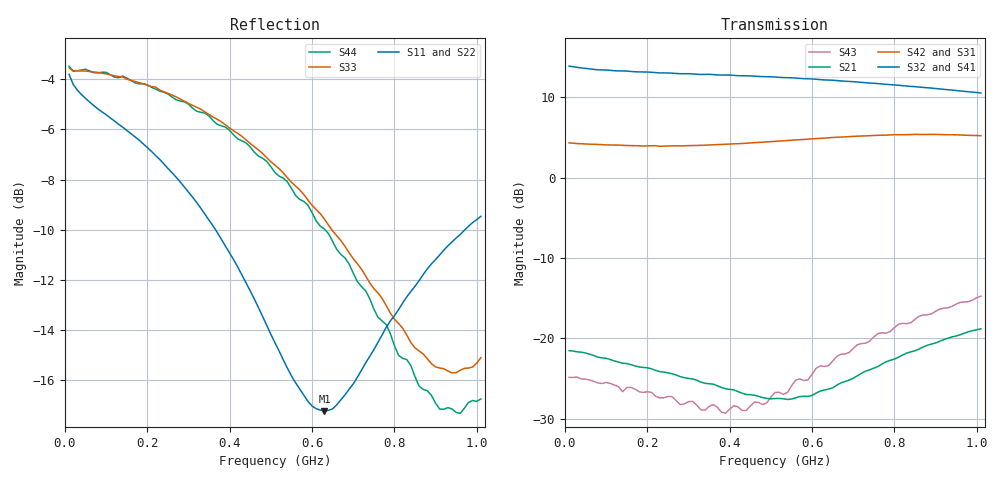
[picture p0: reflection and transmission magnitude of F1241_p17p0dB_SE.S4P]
! Integrated Device Technology
! Corporate Headquarters
! 6024 Silver Creek Valley Road
! San Jose, CA 95138  USA
! Phone:  1-408-284-8200
! Toll Free:  1-800-223-1366
! Webpage:  http://www.idt.com/
! Timing and RF Division
! 515 Groton Road, Suite 102
! Westford, MA 01886-6024
! Device:  F1241
! Description: Dual Intermediate Frequency Digital Variable Gain Amplifier
! Frequency:  10.0 -  500.00 MHz
! Package:  5x5 mm QFN Plastic Package: 32 pin
! Ports:  8 RF, 20 DC
!  Pin  1  = GA3  Pin 17  = RF OUT_B+
!  Pin  2  = GA4  Pin 18  = RF OUT_B-
!  Pin  3  = GA5  Pin 19  = STBY_B
!  Pin  4  = ISET_A  Pin 20  = Ground
!  Pin  5  = ISET_B  Pin 21  = Ground
!  Pin  6  = GB5  Pin 22  = STB_A
!  Pin  7  = GB4  Pin 23  = RF OUT_A-  = Port 4
!  Pin  8  = GB3  Pin 24  = RF OUT_A+  = Port 3
!  Pin  9  = GB2  Pin 25  = NO CONNECT
!  Pin 10  = GB1  Pin 26  = NO CONNECT
!  Pin 11  = RF IN_B+  Pin 27  = VCC
!  Pin 12  = RF IN_B-  Pin 28  = Ground
!  Pin 13  = Ground  Pin 29  = RF IN_A-  = Port 2
!  Pin 14  = VCC  Pin 30  = RF IN_A+  = Port 1
!  Pin 15  = NO CONNECT  Pin 31  = GA1
!  Pin 16  = NO CONNECT  Pin 32  = GA2
! State:  3
! Gain State:  17.0 dB
! Voltages:  Vcc = +5.00 Volts  Icc approximately 160.0 mA or 80 mA per channel.
! Data:  The device was measured on a custom evaluation board which has
!  individual transmission lines to the RF pins.  Data was collected
!  using a calibrated network analyzer.  The evaluation board was
!  de-embedded using a port reference technique.
!  The reference plane is the edge of the package pin.
!  Only Channel A was measured.
!  This data is in single-ended operation.  If your needs are balanced
!  or differential S-parameters then this file needs to be used a
!  linear simulator.
! Misc:  Lot Code  160028MY
!  Action Tracker AT004
! Date Measured:  2014-08-14
! Date:  2014-08-28  MJV
! Note:
!  Integrated Device Technology supplies this data as a sample of measured
!  data at the package pin for this product.  Your particular data for this
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# Hz S dB R 50
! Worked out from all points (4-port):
!   101 points, 10 MHz to 1.01 GHz, reference 50 ohm
!   strongest paths, dB at 10 MHz, 260 MHz, 510 MHz, 760 MHz, 1.01 GHz:
!     S32: 13.8, 13.0, 12.5, 11.7, 10.5
!     S41: 13.9, 12.9, 12.3, 11.5, 10.2
!     S42: 4.3, 3.9, 4.5, 5.3, 5.2
!     S31: 4.3, 3.8, 4.2, 5.0, 5.0
!     S21: -21.5, -24.4, -27.5, -23.5, -18.8
!     S43: -24.8, -27.2, -26.7, -19.4, -14.7
!   lowest |S11| = -17.2 dB at 630 MHz (marker M1), VSWR 1.32, Z = 39.5 - j6.4 ohm
!   |S11| at or under -10 dB: 365.3 MHz to 971.5 MHz (606.2 MHz wide, 90.7 % of centre)
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1e7  -3.80 -10.6  -21.51 7.3  -49.03 37.8  -23.74 6.1
     -21.52 7.1  -3.81 -10.5  -23.75 5.8  -49.10 38.0
     4.31 4.0  13.85 -174.8  -3.54 -7.1  -24.91 17.0
     13.86 -174.8  4.32 4.1  -24.84 16.2  -3.47 -7.3
5e7  -4.76 -13.2  -21.88 -11.6  -43.82 55.2  -24.08 -2.8
     -21.82 -11.4  -4.79 -12.9  -24.02 -2.7  -44.01 55.5
     4.19 -5.1  13.58 172.5  -3.67 -5.3  -25.29 -8.2
     13.57 172.2  4.17 -5.1  -25.06 -6.9  -3.60 -5.4
2.6e8  -7.73 -40.5  -24.47 -48.6  -31.37 54.2  -24.05 -7.2
       -24.39 -51.2  -7.69 -38.6  -24.07 -7.5  -31.40 53.9
       3.81 -24.4  12.98 145.0  -4.63 -21.0  -26.41 -60.3
       12.90 144.3  3.94 -24.1  -27.22 -58.4  -4.71 -20.3
4.6e8  -12.78 -76.1  -27.44 -99.8  -26.90 35.7  -23.10 -15.6
       -27.06 -105.4  -12.82 -72.7  -22.99 -15.5  -26.85 34.7
       4.05 -40.6  12.61 120.5  -6.69 -37.3  -25.37 -124.9
       12.48 119.5  4.34 -41.2  -27.91 -133.5  -6.91 -35.6
6.3e8  -17.24 -144.6  -27.74 -168.9  -24.86 18.5  -22.49 -27.4
       -26.41 -176.4  -17.61 -141.0  -22.23 -27.5  -24.68 16.9
       4.58 -56.8  12.14 99.3  -9.58 -55.2  -21.43 -178.3
       11.97 98.2  4.91 -58.8  -23.48 161.5  -9.98 -50.5
8e8  -13.44 154.1  -23.49 136.1  -23.66 2.0  -22.36 -41.8
     -22.56 131.9  -13.59 154.5  -22.00 -41.8  -23.51 -0.5
     5.06 -76.8  11.52 78.2  -13.58 -82.3  -17.89 139.8
     11.28 77.4  5.33 -79.6  -18.65 126.0  -14.64 -78.1
1.01e9  -9.47 128.1  -19.31 95.5  -22.92 -15.9  -23.08 -58.7
        -18.80 93.0  -9.56 129.0  -22.52 -58.7  -22.74 -19.2
        4.97 -105.0  10.51 52.9  -15.12 -144.1  -14.60 100.8
        10.24 52.2  5.20 -108.4  -14.74 87.7  -16.77 -146.3
